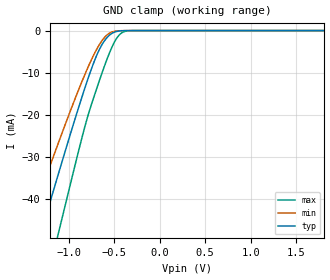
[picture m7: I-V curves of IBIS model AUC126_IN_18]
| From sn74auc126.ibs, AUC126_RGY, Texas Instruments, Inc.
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[Model]   AUC126_IN_18
Model_type  Input
Vinl=0.5775
Vinh=1.2675
| variable   typ   min   max
C_comp   2.33pF   1.89pF   2.69pF
[Temperature Range]   40   100   -40
| Ambient temperature   25   85   -40
[Voltage range]   1.8   1.65   1.95
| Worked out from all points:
|   GND clamp passes 1 mA (typ) near -0.55 V on its own axis
[GND Clamp]
| AUC126_IN_18
|   Voltage   I(typ)   I(min)   I(max)
-3.6V     -222.3mA   -186mA     -267.4mA
-1.475V   -61.14mA   -48.83mA   -80.75mA
-1.43V    -57.76mA   -46.04mA   -76.74mA
-1.295V   -47.69mA   -37.76mA   -64.7mA
-1.1V     -33.32mA   -26.09mA   -47.29mA
-830mV    -14.31mA   -10.95mA   -23.64mA
-680mV    -5.361mA   -4.028mA   -13.09mA
-560mV    -1.272mA   -753.1uA   -5.827mA
-485mV    -290.6uA   -140.1uA   -2.305mA
-420mV    -55.81uA   -26.71uA   -608.5uA
-300mV    -1.501uA   -987.4nA   -11.88uA
1.8V      203.2pA    297.2pA    235.5pA
